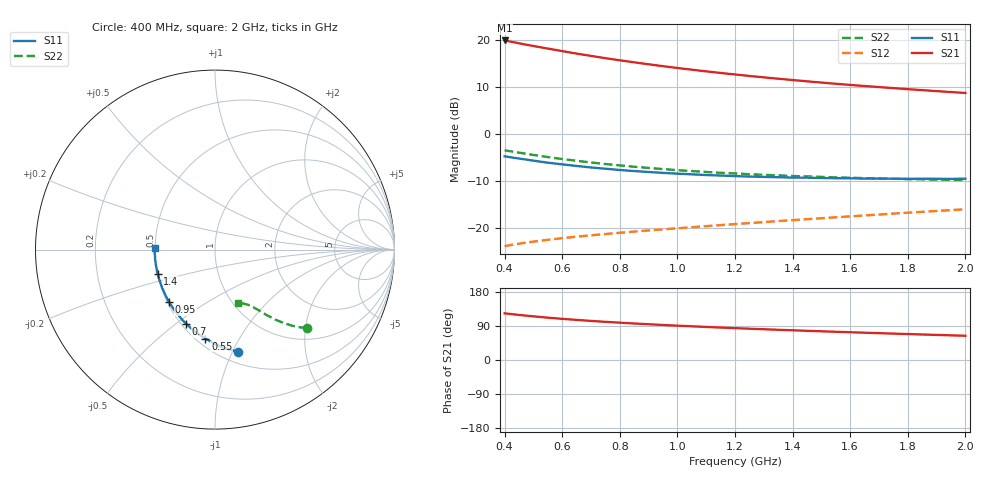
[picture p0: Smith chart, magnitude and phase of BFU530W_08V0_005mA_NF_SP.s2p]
! Filename:  P:\Prog\Test\Noise\ATS_data\Testdata_Net\06 Compressed Noise after Statistics\BFU530W_APM2013_09_A05_08p0V_005mA_NF_CM01_D.sf
! Date/Time: Tue 26/Mar/2013 18:06:03
! BFU530W_APM2013_09_A05_08p0V_1to25mA_NF_CM01_Bias4_R.sf
! Noise Parameter Data File
! BFU530W_APM2013_09_A05_08p0V_1to25mA_NF_CM01
! Date/time: Thu Mar 21 21:44:48 2013
! VAR V_out= 8.000000
! VAR I_out= 4.995000
! VAR V_in= 0.810500
! VAR I_in= 0.050110
! Device data file deembeded for feedlines and parallel
! Original file: \06 Compressed Noise after Statistics\BFU530W_APM2013_09_A05_08p0V_005mA_NF_CM01_R.sf
! Feed-files: PR019V01_070313_Feed1.s2p, PR019V01_070313_Feed2.s2p
! Parallel-file: PR019V01_070313_Par.s2p
# MHz S MA R 50
!  Freq-MHz  S11-mag  S11-arg  S21-mag  S21-arg  S12-mag  S12-arg  S22-mag  S22-arg
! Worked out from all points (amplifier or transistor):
!   37 points, 400 MHz to 2 GHz, reference 50 ohm
!   highest |S21| = 19.9 dB at 400 MHz (marker M1)
!   |S21| within 3 dB of that: start of sweep to 671.5 MHz
!   unconditionally stable (mu >= 1): 1.785 GHz to end of sweep
!   at 500 MHz: K = 0.50, MSG = 20.8 dB, |S12| = -22.8 dB
!   at 1.1 GHz: K = 0.85, MSG = 16.4 dB, |S12| = -19.5 dB
!   at 2 GHz: K = 1.02, MAG = 11.6 dB, |S12| = -15.9 dB
!   lowest NFmin = 0.58 dB at 420 MHz
!   S11 on the Smith chart (normalised r, x): 400 MHz: 0.61, -1.05; 550 MHz: 0.55, -0.73; 700 MHz: 0.53, -0.55; 950 MHz: 0.51, -0.35; 1.4 GHz: 0.50, -0.15; 2 GHz: 0.50, +0.01
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400  0.5828 -77.5  9.893 123.2  0.06476 56.7  0.6746 -40.4
420  0.5697 -80.2  9.623 121.4  0.0665 56.1  0.6592 -41.4
440  0.5573 -83.0  9.366 119.8  0.06809 55.5  0.6441 -42.3
480  0.5351 -88.0  8.863 116.7  0.07101 54.5  0.6163 -43.9
500  0.5238 -90.5  8.634 115.2  0.07239 54.1  0.6025 -44.6
550  0.4984 -96.1  8.112 111.7  0.07559 53.5  0.5719 -46.3
600  0.4783 -101.5  7.625 108.6  0.07873 52.9  0.5448 -47.6
650  0.4602 -106.4  7.176 105.8  0.08167 52.5  0.5223 -48.8
700  0.4435 -111.2  6.781 103.1  0.08444 52.4  0.5012 -50.0
750  0.4301 -115.5  6.415 100.8  0.08712 52.3  0.4822 -50.8
800  0.4168 -119.7  6.09 98.5  0.08984 52.4  0.4667 -51.7
850  0.4062 -123.8  5.794 96.3  0.09249 52.4  0.4511 -52.4
950  0.3884 -131.0  5.277 92.4  0.09771 52.9  0.4265 -53.8
1050  0.3749 -137.6  4.841 88.9  0.1029 53.4  0.406 -54.9
1100  0.3686 -140.7  4.648 87.2  0.1056 53.6  0.3975 -55.5
1200  0.3592 -146.6  4.308 84.1  0.1111 54.2  0.3831 -56.7
1300  0.3522 -152.0  4.013 81.2  0.1166 54.8  0.3703 -57.7
1400  0.3463 -157.1  3.759 78.4  0.1224 55.3  0.3602 -58.8
1500  0.3427 -161.7  3.534 75.7  0.1282 55.8  0.3521 -60.1
1650  0.3383 -168.2  3.247 72.0  0.1372 56.5  0.3416 -61.9
1750  0.3372 -172.2  3.086 69.6  0.1436 56.9  0.3365 -63.1
2000  0.337 178.6  2.741 64.0  0.1596 57.6  0.3267 -66.7
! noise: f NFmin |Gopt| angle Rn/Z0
400  0.6041  0.2011  30.87  0.1103
460  0.6229  0.1805  37.66  0.1054
600  0.6392  0.172  43.63  0.1121
800  0.6834  0.1868  62.02  0.1018
1000  0.7107  0.1968  76.48  0.1002
1200  0.7535  0.2027  92.49  0.0941
1400  0.7835  0.2101  113.7  0.0843
1600  0.7478  0.2399  122  0.0789
1800  0.8135  0.2745  139.3  0.0664
2000  0.8545  0.3114  154.4  0.0551
